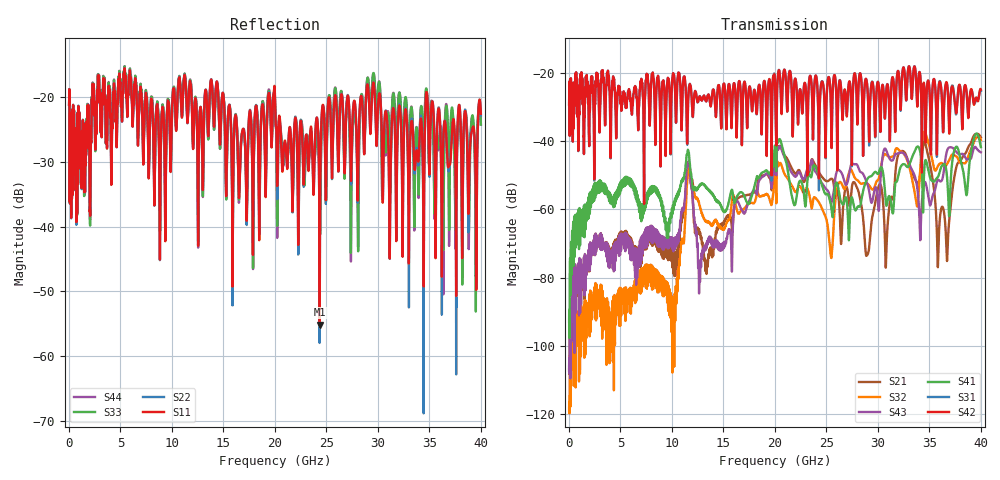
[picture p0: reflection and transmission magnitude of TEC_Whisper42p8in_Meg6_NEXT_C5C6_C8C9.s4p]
! Tyco Electronics Strada Whisper System
! NEXT_C5C6-C8C9
!! SYSTEM DESCRIPTION: Daughtercard-Connector-Backplane-Connector-Daughtercard
!! PCB DESCRIPTION: BP: 250mil, 26 lyrs, Megtron6, bottom layer route, no stub, 6-9-6mil 30" traces; DC: 150mil, 16 lyrs, Megtron6, bottom layer route, no stub, 6-9-6mil 5" traces
!! CONNECTOR DESCRIPTION: STRADA Whisper, Right Angle Receptacle to Vertical Header
!! MODEL DESCRIPTION: Tyco Electronics System 4-port S-parameter
!! MODEL STATUS: Developmental
!! MODEL GEOMETRY: Channel Model
!! MODEL FREQUENCY RANGE: DC to 40 GHz in 10 MHz frequency steps
!! MODEL EDGE RATE LIMITATION: 12.5 ps (Using conservative 0.5/Fmax rule of thumb)
!! TIME-DOMAIN TRANSFORM CAUTIONS:
!! 1.) Do not simulate transient edge rates faster than the number listed above.  Edge rates faster than this number
!!  contain significant spectral content at frequencies above the model's highest frequency.
!! 2.) Even when simulating edge rates that are slower than the number listed above, be aware that the best time
!!  resolution possible with a direct iFFT is (1 / 2Fmax).  As a result, time resolution is typically not adequate
!!  for most time-domain simulations unless tricks such as windowing are used to minimize leakage and aliasing.
!! 3.) Because the model has a uniform frequency step, a direct iFFT will result in an impulse that that has a time
!!  length given by either (1 / Fstep) or (1 / 2Fstep), depending on the transform being used.  Care has been taken
!!  in selecting the frequency step to ensure a settled impulse response for the model.  Therefore, convolution with
!!  the model's impulse response should present no issues.  However, if directly concatenating s-parameter models
!!  in the frequency domain a user must either interpolate necessary interim frequencies or complete impulse response
!!  zero-padding.  Impulse response zero-padding is more difficult, but more accurate.
!! PORT DEFINITIONS:
!! Port  1  ----->  Side A  C8  C5  Side A  <-----  Port  2
!! Port  3  ----->  Side A  C9  C6  Side A  <-----  Port  4
! Created Wed Apr 27 13:54:01 2011
# hz S ma R 50
! 4 Port Network Data from SP1.SP block
! freq  magS11  angS11  magS12  angS12  magS13  angS13  magS14  angS14
!  magS21  angS21  magS22  angS22  magS23  angS23  magS24  angS24
!  magS31  angS31  magS32  angS32  magS33  angS33  magS34  angS34
!  magS41  angS41  magS42  angS42  magS43  angS43  magS44  angS44
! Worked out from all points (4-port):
!   4000 points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, 10 MHz to 40 GHz, reference 50 ohm
!   strongest paths, dB at 10 MHz, 10.01 GHz, 20.01 GHz, 30.01 GHz, 40 GHz:
!     S42: -29.2, -22.6, -23.6, -22.7, -24.9
!     S31: -29.3, -22.6, -23.1, -22.6, -25.3
!     S41: -92.9, -60.3, -41.3, -49.6, -41.7
!     S43: -106.8, -68.8, -43.3, -58.3, -43.2
!     S32: -118.9, -87.9, -47.2, -51.4, -39.7
!     S21: -107.2, -72.0, -42.7, -53.8, -38.9
!   lowest |S11| = -55.1 dB at 24.35 GHz (marker M1), VSWR 1.00, Z = 50 + j0.175 ohm
!   |S11| at or under -10 dB: start of sweep to end of sweep
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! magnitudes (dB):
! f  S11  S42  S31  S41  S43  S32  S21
! 10 MHz  -21.2  -29.2  -29.3  -92.9  -106.8  -118.9  -107.2
! 2.98 GHz  -19.4  -35.7  -35.6  -52.5  -68.0  -83.7  -68.1
! 24.35 GHz  -55.1  -29.6  -29.5  -50.9  -51.2  -58.3  -49.5
! 28.97 GHz  -18.1  -24.1  -24.0  -51.1  -52.5  -52.4  -73.3
! 34.56 GHz  -24.9  -28.0  -28.4  -46.2  -52.0  -37.2  -40.2
! 36.72 GHz  -28.6  -23.3  -23.6  -50.7  -42.7  -46.6  -74.9
! 40 GHz  -22.6  -24.9  -25.3  -41.7  -43.2  -39.7  -38.9
